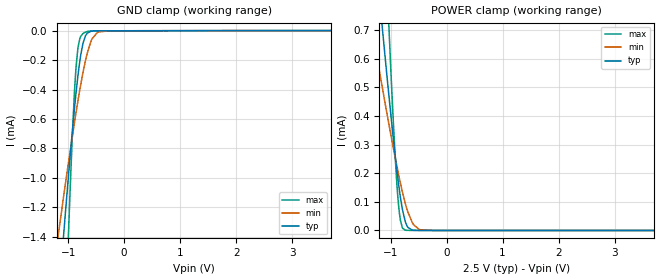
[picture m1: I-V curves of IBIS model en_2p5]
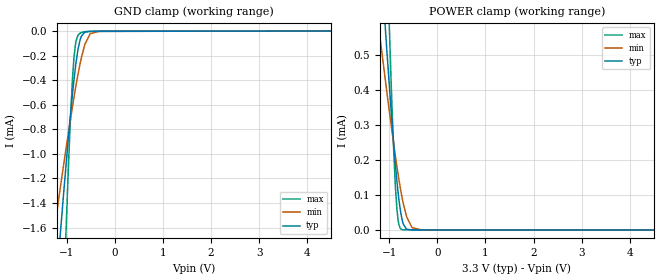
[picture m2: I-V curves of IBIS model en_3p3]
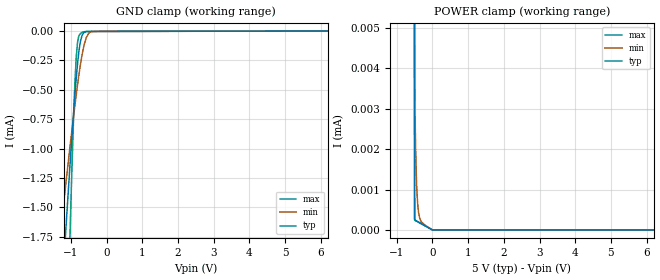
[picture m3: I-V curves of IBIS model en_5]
|Texas Instruments Incorporated
| High-Performance, 8000 VPK Reinforced Dual Channel Digital Isolator
| Marketing part#   Digital Voltage Range   Package-type   #pins
| ISO7821FDW   2.25V-5.5V   SOIC   16
| ISO7821FDWW   2.25V-5.5V   SOIC   16
[IBIS Ver]   4.1
[File name]   iso7821f.ibs
[File Rev]   1.1
[Date]   1/5/2016
[Source]
| Texas Instruments Incorporated.
| Analog-eLab Design Center, HPA
| 12500 TI Blvd
| Dallas, TX -75243
[Notes]   Revision History:
| Rev 1.1: 1/5/2016
| - Add DWW package component and EN buffer model
| Rev 1.0: 7/1/2015
| - Initial version of the model
| - Model generated from simulations in TISPICE
| - Model matched to SPICE simulation
| - C_comp although listed in numerical order of value are
|   obtained from varying PVT conditions. For PVT conditions for
|   each specific value refer the buffer description under
|   respective [Model]. IBIS model user is responsible for using
|   appropriate C_comp to simulate for Signal Integrity.
| - This is relative part of ISO7841F.
|* EXCEPTION:   *
|* - For en_* models there will be leakage current in GROUND clamp  *
|*   because of a resistor(RH2) connected to pad.   *
|* - For in_* models there will be leakage current in POWER clamp   *
|*   because of a resistor(RH2) connected to pad.   *
[Disclaimer]
| This model is designed as an aid for customers of Texas Instruments.
| TI and its licensors and suppliers make no warranties, either expressed
| or implied, with respect to this  model, including the warranties of
| merchantability or fitness for a particular purpose. The model is
| provided solely on an "as is" basis. The entire risk as to its quality
| and performance is with the customer.
[Copyright]
(C) Copyright 2015 Texas Instruments Incorporated.All rights reserved.
|   ISO7821FDW
[Component]   ISO7821FDW
[Manufacturer]   TI
[Package]   |16 SOIC - DW package
|   typ   min   max
R_pkg   0.1398   0.1249   0.1793
L_pkg   2.180nH   1.9245nH   2.8571nH
C_pkg   0.4206pF   0.2145pF   0.6128pF
[Pin]  signal_name   model_name   R_pin   L_pin   C_pin
1   GND1   GND   0.0970   2.2582nH   0.6389pF
2   NC   NC   0.1057   2.1519nH   0.3071pF
3   VCC1   POWER   0.1289   1.9955nH   0.2145pF
4   OUTA   OUT   0.1262   1.9475nH   0.6128pF
5   INB   IN   0.1249   1.9265nH   0.3667pF
6   NC   NC   0.1404   2.1876nH   0.4324pF
7   GND1   GND   0.1781   2.8364nH   0.4590pF
8   NC   NC   0.0822   2.4395nH   0.4450pF
9   GND2   GND   0.1013   2.4407nH   0.4093pF
10   NC   NC   0.1793   2.8571nH   0.5272pF
11   NC   NC   0.1288   1.9962nH   0.5084pF
12   OUTB   OUT   0.1262   1.9440nH   0.3263pF
13   INA   IN   0.1250   1.9245nH   0.3778pF
14   VCC2   POWER   0.1405   2.1861nH   0.3810pF
15   NC   NC   0.0827   2.0901nH   0.7509pF
16   GND2   GND   0.0975   2.2691nH   0.6744pF
|   IS07821FDWW
[Component]   IS07821FDWW
[Manufacturer]   TI
[Package]   |16 SOIC - DWW package
|   typ   min   max
R_pkg   0.2986   0.2007   0.3729
L_pkg   6.1920nH   5.7068nH   6.9814nH
C_pkg   0.3776pF   0.0527pF   0.7658pF
[Pin]  signal_name   model_name   R_pin   L_pin   C_pin
1   VCC1   POWER   0.2515   6.9814nH   0.7658pF
2   GND1   GND   0.2414   6.4743nH   0.4827pF
3   NC   NC   0.3404   6.2419nH   0.3712pF
4   EN1   EN   0.2997   5.8575nH   0.3661pF
5   OUTA   OUT   0.3048   5.7068nH   0.3697pF
6   INB   IN   0.3229   5.9972nH   0.3885pF
7   NC   NC   0.3729   6.6301nH   0.3885pF
8   GND1   GND   0.2162   5.8346nH   0.4827pF
9   GND2   GND   0.2007   6.5823nH   0.5517pF
10   NC   NC   0.3456   6.8632nH   0.3887pF
11   OUTB   OUT   0.3109   6.1891nH   0.3704pF
12   INA   IN   0.2997   5.7473nH   0.3669pF
13   EN2   EN   0.3032   5.8251nH   0.3710pF
14   NC   NC   0.3351   6.1684nH   0.0527pF
15   GND2   GND   0.2007   5.7509nH   0.5517pF
16   VCC2   POWER   0.2768   6.8945nH   0.0527pF
|   Model Selectors
[Model Selector] EN
en_2p5   2.5V digital Input
en_3p3   3.3V digital Input
en_5   5.0V digital Input
[Model Selector] IN
in_2p5   2.5V digital Input
in_3p3   3.3V digital Input
in_5   5.0V digital Input
[Model Selector] OUT
out_2p5   2.5V digital 3-state
out_3p3   3.3V digital 3-state
out_5   5.0V digital 3-state
| Models and submodels in the file (9): en_2p5 (Input), en_3p3 (Input), en_5 (Input), in_2p5 (Input), in_3p3 (Input), in_5 (Input), out_2p5 (3-state), out_3p3 (3-state), out_5 (3-state)
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|   en_2p5 Model
[Model]   en_2p5
Model_type   Input
Vinl = 0.75
Vinh = 1.75
|   typ   min   max
|   (nom PVT)   (fast PVT)   (slow PVT)
C_comp   3.303e-15   3.281e-15   1.151e-13
[Model spec]
|subparameter
Vinl   0.75   0.675   0.825
Vinh   1.75   1.575   1.925
| Where nom  PVT is Nominal Process, 2.5V, 27C
|   Fast PVT is Strong Process,  2.75V, -55C
|   Slow PVT is Weak Process,   2.25V, 150C
[Voltage Range]   2.5   2.25   2.75
|Junction Temperature
[Temperature Range]   27   150   -55
[Power Clamp Reference]   2.5   2.25   2.75
[GND Clamp Reference]   0   0   0
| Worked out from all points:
|   GND clamp passes 1 mA (typ) near -1.00 V on its own axis
|   POWER clamp passes 1 mA (typ) near -1.29 V on its own axis
[GND Clamp]
|   Voltage   I(typ)   I(min)   I(max)
-2.5V     -8.647mA   -5.195mA   -19.82mA
-1.224V   -2.083mA   -1.519mA   -3.979mA
-1.065V   -1.316mA   -1.086mA   -2.148mA
-1.001V   -1.021mA   -917uA     -1.46mA
-891.2mV  -548.7uA   -636.9uA   -451.9uA
-857.5mV  -419.8uA   -554.9uA   -246.1uA
-825.3mV  -308.5uA   -479.2uA   -120.6uA
-789.5mV  -203.1uA   -398.8uA   -52.86uA
-691mV    -36.17uA   -205.8uA   -10.4uA
-575mV    -3.575uA   -57.61uA   -2.24uA
-250mV    -1.373uA   -1.462uA   -1.451uA
5V        0A         0A         0A
[POWER Clamp]
|   Voltage   I(typ)   I(min)   I(max)
-2.5V     3.622mA    2.076mA    7.967mA
-1.351V   1.129mA    727.2uA    2.224mA
-1.196V   807.1uA    553.5uA    1.48mA
-1.053V   516.7uA    396.2uA    813.3uA
-990.2mV  394.3uA    329.2uA    537.7uA
-924.3mV  272.7uA    261.2uA    278.2uA
-874.8mV  189uA      212.4uA    126.7uA
-822.5mV  113uA      163.7uA    33.56uA
-740mV    33.03uA    96.34uA    1.225uA
-612.5mV  1.036uA    27.5uA     297.8nA
-486.3mV  250nA      2.81uA     235.3nA
5V        0A         0A         0A
|   en_3p3 Model
[Model]   en_3p3
Model_type   Input
Vinl = 0.99
Vinh = 2.31
|   typ   min   max
|   (nom PVT)   (fast PVT)   (slow PVT)
C_comp   3.303e-15   3.281e-15   1.158e-13
[Model spec]
|subparameter
Vinl   0.99   0.891   1.089
Vinh   2.31   2.079   2.541
| Where nom  PVT is Nominal Process, 3.3V, 27C
|   Fast PVT is Strong Process,  3.63V, -55C
|   Slow PVT is Weak Process,   2.97V, 150C
[Voltage Range]   3.3   2.97   3.63
|Junction Temperature
[Temperature Range]   27   150   -55
[Power Clamp Reference]   3.3   2.97   3.63
[GND Clamp Reference]   0   0   0
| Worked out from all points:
|   GND clamp passes 1 mA (typ) near -1.00 V on its own axis
|   POWER clamp passes 1 mA (typ) near -1.29 V on its own axis
[GND Clamp]
|   Voltage   I(typ)   I(min)   I(max)
-3.3V     -12.85mA   -7.552mA   -29.96mA
-1.251V   -2.215mA   -1.593mA   -4.295mA
-1.213V   -2.028mA   -1.488mA   -3.846mA
-1.063V   -1.305mA   -1.079mA   -2.122mA
-980.4mV  -927.6uA   -862.8uA   -1.246mA
-926mV    -691uA     -723.5uA   -729.1uA
-849.8mV  -392.1uA   -536.5uA   -209.7uA
-808.2mV  -255.7uA   -440.3uA   -80.89uA
-697.3mV  -41.71uA   -216.6uA   -11.76uA
-511.2mV  -2.293uA   -20.49uA   -2.098uA
-330mV    -1.815uA   -2.199uA   -1.916uA
6.6V      0A         0A         0A
[POWER Clamp]
|   Voltage   I(typ)   I(min)   I(max)
-3.3V     5.384mA    3.032mA    12.02mA
-1.242V   901.1uA    604.2uA    1.697mA
-1.198V   810uA      555uA      1.487mA
-1.049V   509.1uA    392uA      796uA
-965.9mV  348.5uA    303.8uA    437.1uA
-878.8mV  195.5uA    216.3uA    137uA
-842.5mV  140.2uA    181.9uA    60.64uA
-805.2mV  91.77uA    148.5uA    18.16uA
-737.2mV  31.27uA    94.34uA    1.112uA
-526mV    293.6nA    6.522uA    254.6nA
-330mV    164.9nA    232nA      159.7nA
6.6V      0A         0A         0A
|   en_5 Model
[Model]   en_5
Model_type   Input
Vinl = 1.5
Vinh = 3.5
|   typ   min   max
|   (nom PVT)   (fast PVT)   (slow PVT)
C_comp   3.303e-15   3.281e-15   1.164e-13
[Model spec]
|subparameter
Vinl   1.5   1.35   1.65
Vinh   3.5   3.15   3.85
| Where nom  PVT is Nominal Process, 5V, 27C
|   Fast PVT is Strong Process,  5.5V, -55C
|   Slow PVT is Weak Process,   4.5V, 150C
[Voltage Range]   5   4.5   5.5
|Junction Temperature
[Temperature Range]   27   150   -55
[Power Clamp Reference]   5   4.5   5.5
[GND Clamp Reference]   0   0   0
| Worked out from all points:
|   GND clamp passes 1 mA (typ) near -1.00 V on its own axis
[GND Clamp]
|   Voltage   I(typ)   I(min)   I(max)
-5V       -21.84mA   -12.59mA   -51.61mA
-1.304V   -2.48mA    -1.741mA   -4.932mA
-1.155V   -1.749mA   -1.331mA   -3.177mA
-1.128V   -1.616mA   -1.256mA   -2.86mA
-1.029V   -1.148mA   -990.1uA   -1.755mA
-927.5mV  -697.6uA   -727.4uA   -742.8uA
-855mV    -411.2uA   -549.1uA   -234.7uA
-790mV    -205uA     -400.1uA   -54.24uA
-685mV    -32.64uA   -196.1uA   -10.51uA
-567.5mV  -4.417uA   -52.27uA   -3.419uA
-369.5mV  -2.688uA   -3.564uA   -2.84uA
10V       0A         0A         0A
[POWER Clamp]
|   Voltage   I(typ)   I(min)   I(max)
-5V       371.1mA    133.7mA    611.2mA
-1.007V   426.4uA    346.8uA    609.2uA
-500mV    261.7nA    3.784uA    242nA
-491mV    253.9nA    3.115uA    237.6nA
-482mV    247nA      2.562uA    233.3nA
-473mV    240.7nA    2.107uA    228.9nA
-460mV    232.6nA    1.595uA    222.6nA
-432.5mV  217.1nA    909.5nA    209.3nA
-392mV    196.1nA    454.6nA    189.8nA
-306.5mV  153.2nA    197.5nA    148.4nA
-500uV    0A         0A         0A
10V       0A         0A         0A
